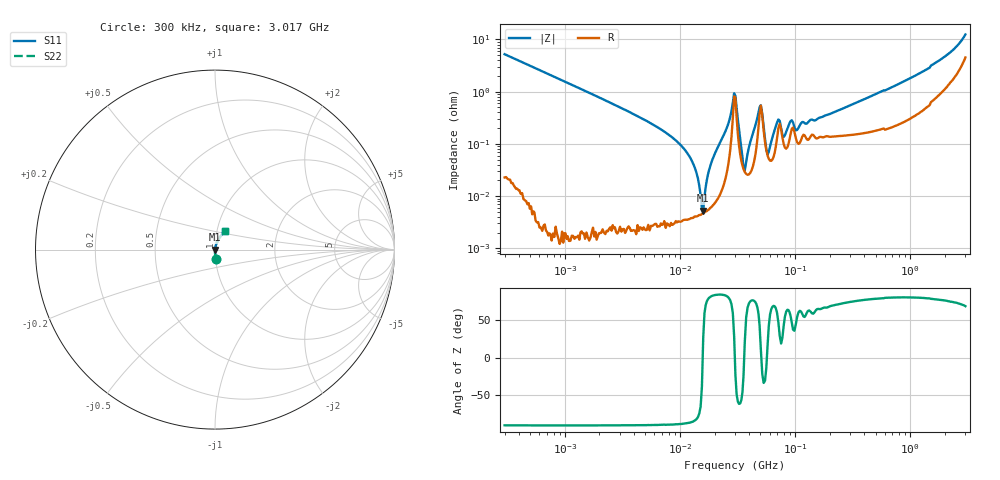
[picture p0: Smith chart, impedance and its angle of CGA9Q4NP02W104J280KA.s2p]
! S-Parameter Data Generated by TDK Corporation
! Copyright(C) 2024 TDK Corporation.
! All Rights Reserved.
! TDK P/N: CGA9Q4NP02W104J280KA (Multilayer Ceramic Chip Capacitor)
! Property: C=100nF
! Size(LxWxT): 5.7x5x2.8mm
! Model Type: s2p (Touchstone File Format Version 1.0)
! Frequency: DC=Yes Start=0.3MHz Stop=3016.958361MHz 374points Log-sweep
! Model Generated on May 28, 2024
! Terms and conditions regarding TDK Simulation Models:
! 1)This simulation model is being provided solely for informational
!  purposes. Please refer to the specifications of the products in
!  terms of detailed characteristics of such products.
! 2)In no event shall TDK Corporation of any of its subsidiaries be
!  liable for any loss or damage arising, directly or indirectly,
!  from any information contained in this simulation model, including,
!  but not limited to loss or damages arising from any inaccuracies,
!  omissions or errors in connection with such information.
! 3)Any and all copyrights on this simulation model are owned by
!  TDK Corporation.  Duplication or redistribution of this simulation
!  model without prior written permission from TDK Corporation
!  is prohibited.
! 4)This simulation model is subject to any modification or change
!  without any prior notice.
! 5)Neither TDK Corporation nor any of its subsidiaries shall make any
!  warranty, express or implied, including but not limited to the
!  correctness, implied warranties of merchantability and fitness for
!  a particular purpose with respect to this simulation models.
! 6)The use of this simulation model shall be deemed to have consented
!  to the terms and conditions hereof.
! Port Assignments:
!  1 ---| |--- 2
! Applicable Conditions:
!  Temperature = 25 degC
!  DC Bias Voltage = 0 V
!  Small Signal Operation
# Hz S MA R 50
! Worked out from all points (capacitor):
!   373 points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, 300 kHz to 3.017 GHz, reference 50 ohm
!   read as one part in series: C = 102 nF near 308.6 kHz
!   lowest |Z| = 5.24 mohm at 15.93 MHz (marker M1)
!   series resonance near 15.77 MHz, so ESL is about 1 nH
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300000  0.05213 -86.8  0.9984 3.0  0.9984 3.0  0.05213 -86.8
1400461  0.0111 -89.3  0.9999 0.6  0.9999 0.6  0.0111 -89.3
6524543  0.002028 -89.1  1 0.1  1 0.1  0.002028 -89.1
1.183796e7  0.0006212 -86.6  1 0.0  1 0.0  0.0006212 -86.6
1.51285e7  0.0001038 -65.0  1 0.0  1 0.0  0.0001038 -65.0
1.593136e7  5.24e-05 26.5  1 -0.0  1 -0.0  5.24e-05 26.5
1.874137e7  0.0004398 81.9  0.9999 -0.0  0.9999 -0.0  0.0004398 81.9
2.585739e7  0.00218 81.3  0.9997 -0.1  0.9997 -0.1  0.00218 81.3
2.956217e7  0.009276 28.9  0.9919 -0.3  0.9919 -0.3  0.009276 28.9
3.032632e7  0.008296 -22.2  0.9923 0.2  0.9923 0.2  0.008296 -22.2
3.567535e7  0.0003603 -23.6  0.9997 0.0  0.9997 0.0  0.0003603 -23.6
3.656965e7  0.0003097 20.5  0.9997 -0.0  0.9997 -0.0  0.0003097 20.5
5.045501e7  0.005483 10.9  0.9946 -0.1  0.9946 -0.1  0.005483 10.9
5.772802e7  0.0006262 16.9  0.9994 -0.0  0.9994 -0.0  0.0006262 16.9
7.161949e7  0.002928 47.3  0.998 -0.1  0.998 -0.1  0.002928 47.3
7.964712e7  0.001355 42.5  0.999 -0.1  0.999 -0.1  0.001355 42.5
9.168857e7  0.002754 54.6  0.9984 -0.1  0.9984 -0.1  0.002754 54.6
1.015821e8  0.00182 44.7  0.9987 -0.1  0.9987 -0.1  0.00182 44.7
1.401524e8  0.002927 59.0  0.9985 -0.1  0.9985 -0.1  0.002927 59.0
6.649102e8  0.01164 79.4  0.9979 -0.7  0.9979 -0.7  0.01164 79.4
1.4785e9  0.02876 77.3  0.9941 -1.6  0.9941 -1.6  0.02876 77.3
3.016958e9  0.1185 62.3  0.9508 -6.3  0.9508 -6.3  0.1185 62.3
